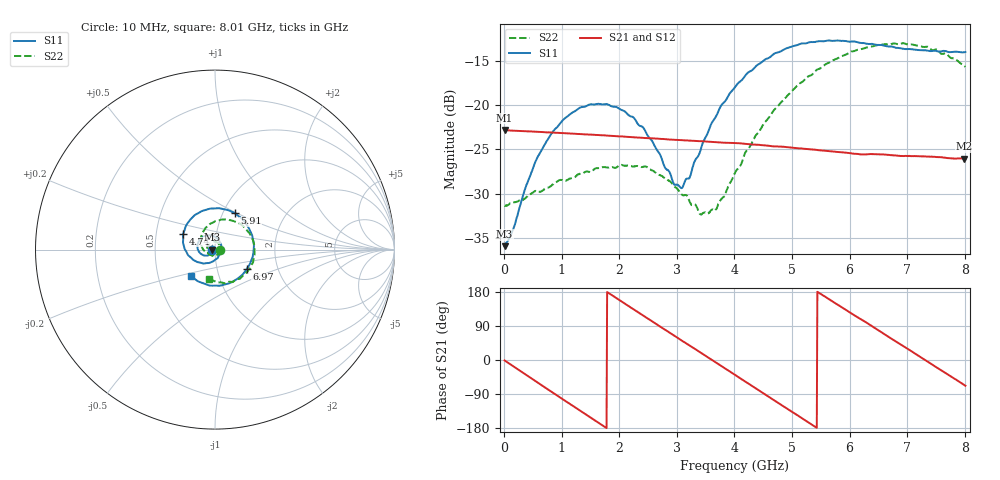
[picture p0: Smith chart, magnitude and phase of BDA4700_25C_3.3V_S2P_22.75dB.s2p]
!Agilent Technologies,E5071B,MY42404982,A.09.10
!Date: Mon Oct 20 18:12:37 2025
!Data & Calibration Information:
!Freq	S11:SOLT2(ON)	S21:SOLT2(ON)	S12:SOLT2(ON)	S22:SOLT2(ON)
# Hz S RI R 50
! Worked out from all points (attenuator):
!   801 points, 10 MHz to 8.01 GHz, reference 50 ohm
!   highest |S21| = -22.82 dB at 10 MHz (marker M1); lowest = -26.0 dB at 7.99 GHz (marker M2)
!   lowest |S11| = -35.9 dB at 10 MHz (marker M3), VSWR 1.03, Z = 48.4 - j0.11 ohm
!   |S11| at or under -10 dB: start of sweep to end of sweep
!   |S22| runs from -32.4 to -13.0 dB; largest |S21 - S12| = 0.00094
!   S11 on the Smith chart (normalised r, x): 10 MHz: 0.97, -0.00; 4.74 GHz: 0.69, +0.13; 5.91 GHz: 1.13, +0.49; 6.97 GHz: 1.38, -0.32; 8.01 GHz: 0.73, -0.22
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1e7  -0.0159 -0.00114  0.0723 -0.00152  0.0723 -0.00161  0.0271 -0.000828
1.5e8  -0.017 -0.00976  0.069 -0.0193  0.069 -0.0193  0.0272 -0.00732
6.1e8  -0.0408 -0.0332  0.0328 -0.0625  0.0328 -0.0625  0.0125 -0.0299
1.01e9  -0.0778 -0.0245  -0.0152 -0.0678  -0.0151 -0.0678  -0.0153 -0.0345
1.35e9  -0.0973 0.00663  -0.0499 -0.047  -0.0499 -0.0471  -0.0368 -0.0181
2.08e9  -0.0501 0.0781  -0.0578 0.0327  -0.0578 0.0327  -0.0298 0.0343
2.42e9  -0.00381 0.0743  -0.0295 0.0582  -0.0295 0.0582  -0.00451 0.0446
2.68e9  0.0242 0.0486  -0.00138 0.0646  -0.00155 0.0645  0.0137 0.0381
2.95e9  0.0345 0.00952  0.0272 0.0576  0.0271 0.0575  0.0262 0.0232
3.09e9  0.0318 -0.0121  0.04 0.0491  0.0396 0.0494  0.0287 0.012
3.41e9  0.00225 -0.0553  0.0589 0.0211  0.059 0.0211  0.0211 -0.0119
3.54e9  -0.0172 -0.0679  0.0617 0.00746  0.0618 0.0074  0.0137 -0.0203
3.69e9  -0.0449 -0.0751  0.0611 -0.00834  0.0612 -0.00849  0.000938 -0.0259
4.01e9  -0.1091 -0.0636  0.0472 -0.0386  0.0473 -0.0385  -0.0318 -0.0262
4.74e9  -0.1763 0.0893  -0.0212 -0.0545  -0.0209 -0.0546  -0.0794 0.0565
5.35e9  -0.0638 0.2177  -0.0554 -0.00867  -0.0554 -0.00893  -0.0157 0.1479
5.91e9  0.1091 0.2033  -0.0377 0.0386  -0.0378 0.0383  0.1106 0.1562
6.68e9  0.2135 -0.0183  0.0256 0.0456  0.0257 0.0455  0.22 -0.00159
6.97e9  0.1759 -0.1095  0.0433 0.0282  0.0433 0.0279  0.2072 -0.0793
7.48e9  0.0303 -0.2005  0.0489 -0.0145  0.0489 -0.0146  0.1036 -0.1777
7.99e9  -0.1306 -0.15  0.0203 -0.0455  0.0204 -0.0456  -0.0271 -0.1645
8.01e9  -0.136 -0.1461  0.0187 -0.0462  0.0189 -0.0462  -0.0319 -0.1614
